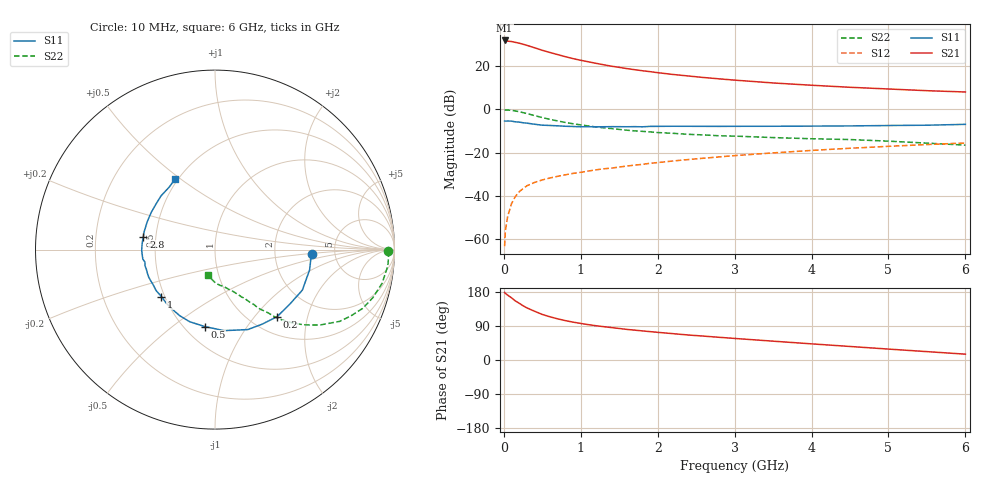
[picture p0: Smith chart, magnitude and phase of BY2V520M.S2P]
! SIEMENS Small Signal Semiconductors
! BFY420
! Si NPN RF SIEGET Grounded Emitter Transistor in MICRO-X
! VCE = 2.5 V  IC = 20 mA
! Common Emitter S-Parameters:  October  1996
# GHz  S  MA  R  50
!  f  S11  S21  S12  S22
! GHz  MAG  ANG  MAG  ANG  MAG  ANG  MAG  ANG
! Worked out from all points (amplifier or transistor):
!   36 points, 10 MHz to 6 GHz, reference 50 ohm
!   highest |S21| = 31.8 dB at 10 MHz (marker M1)
!   |S21| within 3 dB of that: start of sweep to 366.5 MHz
!   unconditionally stable (mu >= 1): 1.97 GHz to end of sweep
!   at 250 MHz: K = 0.30, MSG = 33.3 dB, |S12| = -36.5 dB
!   at 1.4 GHz: K = 0.91, MSG = 23.5 dB, |S12| = -27.1 dB
!   at 6 GHz: K = 1.07, MAG = 10.1 dB, |S12| = -15.5 dB
!   S11 on the Smith chart (normalised r, x): 10 MHz: 3.32, -0.25; 200 MHz: 1.31, -1.32; 500 MHz: 0.62, -0.66; 1 GHz: 0.48, -0.30; 2.8 GHz: 0.43, +0.07; 6 GHz: 0.48, +0.48
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0.01  0.5396 -2.8  38.91 178.4  0.0007 102.4  0.9634 -0.6
0.02  0.5365 -5.1  38.66 175.7  0.0016 87.4  0.9681 -1.7
0.1  0.5365 -24.9  36.75 164.0  0.0067 81.2  0.9497 -11.4
0.15  0.5158 -36.0  35.18 155.8  0.0098 75.2  0.9197 -16.9
0.2  0.5094 -47.1  33.69 149.8  0.0126 71.3  0.8856 -21.7
0.25  0.4917 -57.6  31.83 143.1  0.0149 68.0  0.8417 -26.1
0.3  0.4815 -67.7  29.99 137.5  0.0173 66.3  0.8017 -29.9
0.4  0.4544 -83.6  26.39 128.6  0.0207 62.5  0.7188 -35.8
0.5  0.4325 -97.7  23.06 120.2  0.0236 60.5  0.6481 -40.3
0.6  0.4258 -109.4  20.52 114.0  0.0262 58.6  0.5895 -43.7
0.7  0.4175 -118.1  18.35 108.6  0.0286 58.2  0.5413 -46.4
0.8  0.4083 -126.4  16.42 103.9  0.031 57.4  0.4998 -48.4
1  0.3969 -138.7  13.57 96.5  0.0353 57.1  0.4392 -51.2
1.1  0.3996 -145.2  12.51 93.2  0.0379 57.5  0.4148 -52.9
1.4  0.3999 -157.5  9.906 85.5  0.0442 58.2  0.361 -55.9
1.6  0.3977 -164.1  8.724 80.7  0.0494 57.4  0.3311 -57.9
2.2  0.4084 -179.3  6.389 69.5  0.0646 56.2  0.2805 -63.1
2.8  0.4057 169.7  5.061 59.9  0.0802 53.4  0.2463 -67.8
3.5  0.4083 157.6  4.072 49.7  0.0992 49.0  0.2239 -73.3
4.5  0.4159 141.7  3.235 35.7  0.1269 41.3  0.2015 -82.0
5.5  0.4316 126.2  2.7 22.1  0.1546 32.2  0.1667 -96.0
6  0.452 119.4  2.52 15.4  0.1678 27.5  0.1499 -105.8
